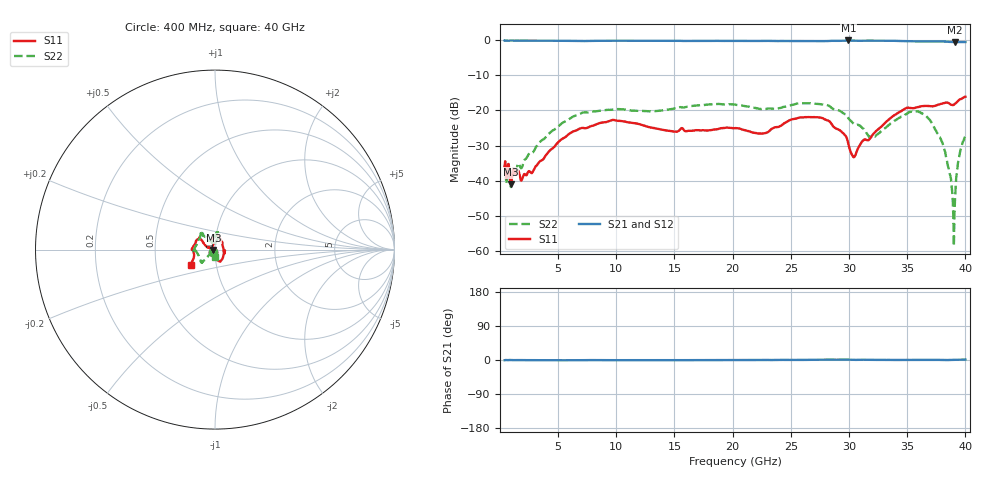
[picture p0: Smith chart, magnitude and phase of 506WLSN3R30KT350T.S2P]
!  American Technical Ceramics  Date:  8/31/2012
!  One Norden Lane
!  Huntington Station,  NY.  11746-2102
!  Tel:  (631) 622-4700  Fax:  (631) 622-4748
!  Part Number  506WLSN3R30KG350T
!  Description:  Ultra-Broadband Inductor
!  Application:  Ultra-broadband DC block decoupling, bias tee
# GHZ S DB R 50
! Freq  |S11|  S11 Ph  |S21|  S21 Ph  |S12|  S12 Ph  |S22|  S22 Ph
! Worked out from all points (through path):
!   801 points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, 400 MHz to 40 GHz, reference 50 ohm
!   highest |S21| = -0.06 dB at 29.95 GHz (marker M1); lowest = -0.5 dB at 39.11 GHz (marker M2)
!   lowest |S11| = -41.0 dB at 944.5 MHz (marker M3), VSWR 1.02, Z = 49.2 - j0.246 ohm
!   |S11| at or under -10 dB: start of sweep to end of sweep
!   |S22| runs from -58.6 to -17.9 dB; largest |S21 - S12| = 0.0058
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0.4  -35.78 -134.8  -0.09 -0.6  -0.08 -0.6  -36.34 -134.3
0.9445  -41.00 -163.7  -0.06 -0.1  -0.06 -0.1  -41.81 -160.4
2.776  -37.70 -118.7  -0.10 -0.4  -0.10 -0.4  -32.10 -145.8
7.033  -24.98 -85.9  -0.21 -0.6  -0.21 -0.6  -20.71 -135.4
9.7555  -22.68 -66.3  -0.13 -0.4  -0.14 -0.5  -19.73 -135.5
13.6165  -25.25 -25.8  -0.15 -0.6  -0.15 -0.6  -20.09 -165.5
20.2  -25.05 -21.5  -0.19 -0.1  -0.19 -0.0  -18.32 -176.4
22.675  -26.54 21.0  -0.19 0.2  -0.20 0.2  -19.60 159.4
26.833  -21.89 92.0  -0.24 0.4  -0.23 0.5  -17.99 126.4
28.2685  -23.02 98.0  -0.21 1.2  -0.21 1.2  -18.68 128.0
29.9515  -29.70 105.5  -0.06 0.9  -0.06 1.0  -22.24 123.4
30.4465  -33.25 143.0  -0.10 0.4  -0.09 0.5  -23.93 126.9
31.882  -27.69 164.1  -0.10 0.5  -0.10 0.6  -27.55 113.5
33.4165  -22.58 150.2  -0.17 0.3  -0.15 0.4  -24.15 96.2
35.3965  -19.33 143.2  -0.30 -0.1  -0.29 0.1  -20.30 83.3
36.832  -18.68 156.0  -0.36 0.3  -0.35 0.4  -22.26 76.1
38.0695  -17.95 176.0  -0.36 0.1  -0.35 0.2  -29.71 87.1
38.614  -18.03 -178.3  -0.46 -0.0  -0.44 0.1  -37.23 103.8
38.911  -18.45 -168.6  -0.50 0.3  -0.50 0.4  -45.33 88.4
39.109  -18.11 -161.0  -0.53 0.6  -0.52 0.7  -45.22 -65.2
39.4555  -16.98 -153.5  -0.51 1.0  -0.50 1.1  -33.33 -83.8
40  -16.07 -147.7  -0.51 1.3  -0.48 1.4  -27.35 -92.7
